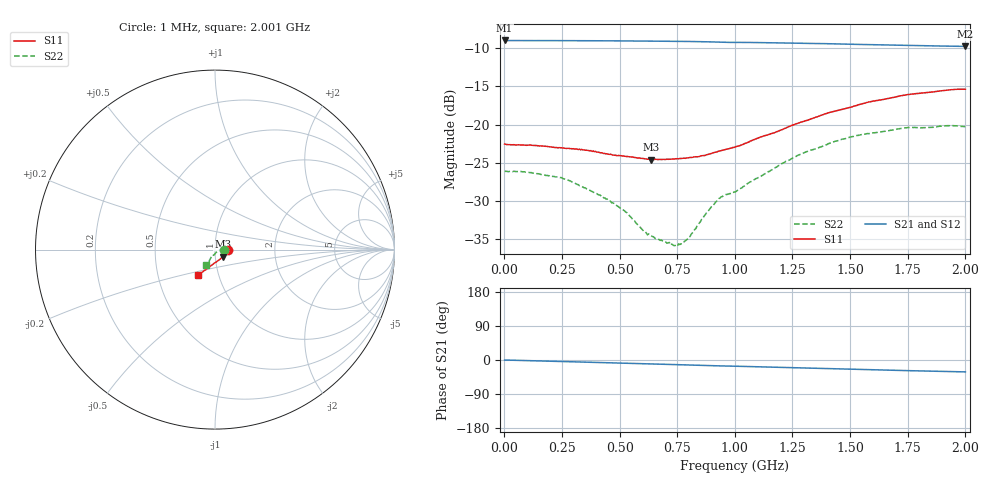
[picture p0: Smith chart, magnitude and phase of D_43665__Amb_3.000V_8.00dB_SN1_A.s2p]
! device id: 43665_
! dir: \\malibu\benchdata\1_engineers\tn_data\43665_75ohm\new\sparar\43665_\amb\3p000v\8p00db
! Serial: 1
! Insertion: A
! Temp: Amb
! VDD: 3.000V
! Attenuation Step: 8.00dB
! IDD: 1.453655e+00mA
! FILE NAME
! DATE 03-27-2009 08:35:19
! CORRECTED  DATA
#  Hz  S  RI  R  75
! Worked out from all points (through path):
!   401 points, 1 MHz to 2.001 GHz, reference 75 ohm
!   highest |S21| = -8.99 dB at 1 MHz (marker M1); lowest = -9.8 dB at 2.001 GHz (marker M2)
!   group delay of S21, straight-line fit = 44.5 ps
!   lowest |S11| = -24.6 dB at 636 MHz (marker M3), VSWR 1.13, Z = 81.5 - j6.58 ohm
!   |S11| at or under -10 dB: start of sweep to end of sweep
!   |S22| runs from -35.9 to -20.1 dB; largest |S21 - S12| = 0.0015
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1000000  0.0745 -0.00095  0.3553 -0.000668  0.3555 -0.000509  0.0497 -0.000697
9.6e7  0.0729 -0.00547  0.3546 -0.00952  0.3547 -0.00957  0.0488 0.0015
2.36e8  0.0693 -0.0134  0.3536 -0.0233  0.3537 -0.0234  0.0451 0.00246
3.36e8  0.0658 -0.0196  0.3524 -0.0333  0.3525 -0.0333  0.0392 0.00274
4.46e8  0.0587 -0.0262  0.3507 -0.0442  0.3507 -0.0443  0.0325 4.69e-05
5.21e8  0.0533 -0.0317  0.3489 -0.0518  0.3491 -0.0519  0.0271 -0.00239
6.11e8  0.0456 -0.0384  0.3466 -0.0605  0.3466 -0.0606  0.019 -0.0057
6.36e8  0.043 -0.0403  0.3459 -0.0631  0.3459 -0.0631  0.0173 -0.00702
6.71e8  0.0402 -0.0432  0.3451 -0.0666  0.345 -0.0666  0.0151 -0.0092
7.41e8  0.0336 -0.0491  0.3429 -0.0737  0.3429 -0.0736  0.0097 -0.0129
7.71e8  0.0306 -0.0516  0.3418 -0.0768  0.3417 -0.0767  0.00682 -0.015
8.06e8  0.0269 -0.0546  0.3404 -0.0803  0.3404 -0.0803  0.00355 -0.0181
8.76e8  0.0182 -0.0605  0.3371 -0.0876  0.3371 -0.0874  -0.00211 -0.0262
9.26e8  0.0116 -0.0655  0.3338 -0.092  0.334 -0.0918  -0.008 -0.0309
9.51e8  0.00913 -0.0673  0.3324 -0.0935  0.3326 -0.0933  -0.0124 -0.0319
1.001e9  0.00336 -0.071  0.3311 -0.0969  0.3312 -0.0967  -0.0169 -0.032
1.211e9  -0.0236 -0.0902  0.322 -0.1162  0.3224 -0.1162  -0.0252 -0.0501
1.336e9  -0.0392 -0.1022  0.3151 -0.1263  0.3157 -0.1264  -0.0314 -0.0607
1.501e9  -0.0583 -0.1157  0.3054 -0.1388  0.3058 -0.1392  -0.0386 -0.0732
1.671e9  -0.0757 -0.128  0.2957 -0.1504  0.2956 -0.1511  -0.043 -0.0805
1.756e9  -0.0825 -0.1341  0.2907 -0.1557  0.2908 -0.1567  -0.0447 -0.0844
2.001e9  -0.096 -0.1408  0.2772 -0.1692  0.276 -0.1701  -0.0496 -0.0831
